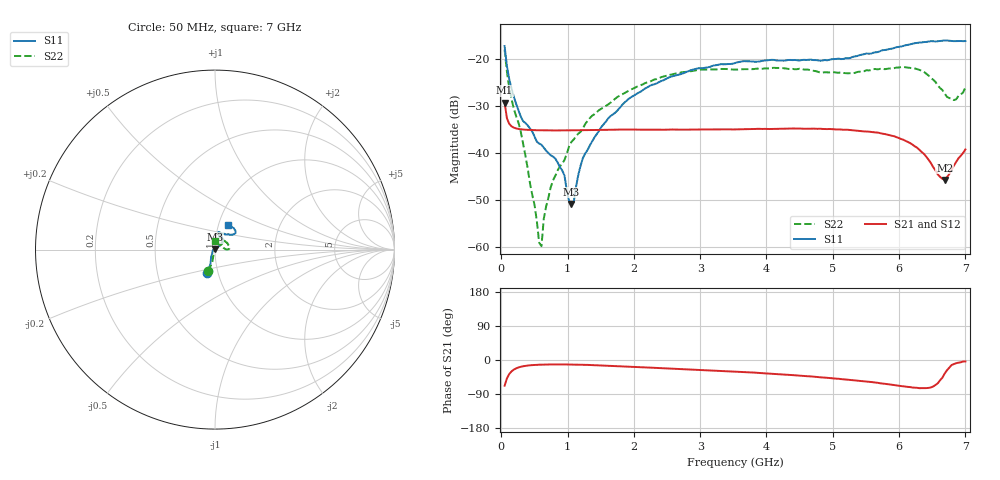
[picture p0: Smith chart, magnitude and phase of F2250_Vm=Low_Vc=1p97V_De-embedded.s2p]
! Integrated Device Technology
! Corporate Headquarters
! 6024 Silver Creek Valley Road
! San Jose, CA 95138  USA
! Phone:  1-408-284-8200
! Toll Free:  1-800-223-1366
! Webpage:  http://www.idt.com/
! Timing and RF Division
! 515 Groton Road, Suite 102
! Westford, MA 01886-6024
! Device:  F2250
! Description: Voltage Variable RF Attenuator
! Frequency:  50.0 -  6000.00 MHz
! Package:  3x3 mm Thin QFN Plastic Package: 16 pin
! Ports:  2 RF, 3 DC
!  Pin  1  = GND
!  Pin  2  = NC
!  Pin  3  = RF1  = Port 1
!  Pin  4  = NC
!  Pin  5  = GND
!  Pin  6  = GND
!  Pin  7  = GND
!  Pin  8  = GND
!  Pin  9  = NC
!  Pin 10  = RF2  = Port 2
!  Pin 11  = NC
!  Pin 12  = GND
!  Pin 13  = GND
!  Pin 14  = VCNTRL
!  Pin 15  = VDD
!  Pin 16  = VMODE
! Vcntrl:  1.970 Volts
! Vmode:  +0.000 Volts
! Vdd:  +3.30  Volts
! Current:  1.185 mA
! Data:  The device was measured on a the F2250 evaluation board which has
!  individual transmission lines to the RF pins.  Data was collected
!  using a calibrated network analyzer.  The evaluation board was
!  de-embedded using a TRL calibration technique.
!  The reference plane is the edge of the package pin.
! Misc:  SN 10
!  Action Tracker AT0258
! Date Measured:  2014-11-26
! Date:  2015-10-15  MJV
! Note:
!  Integrated Device Technology supplies this data as a sample of measured
!  data at the package pin for this product.  Your particular data for this
!  product may vary.
!  Data was taken at 25 degrees C.
!  Integrated Device Technology reserves the right to change this data at anytime.
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# GHz S dB R 50
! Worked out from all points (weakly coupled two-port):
!   201 points, 50 MHz to 7 GHz, reference 50 ohm
!   highest |S21| = -29.23 dB at 50 MHz (marker M1); lowest = -45.8 dB at 6.687 GHz (marker M2)
!   lowest |S11| = -50.9 dB at 1.058 GHz (marker M3), VSWR 1.01, Z = 49.8 + j0.242 ohm
!   |S11| at or under -10 dB: start of sweep to end of sweep
!   |S22| runs from -59.9 to -17.9 dB; largest |S21 - S12| = 5.7e-05
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0.05  -17.18 -108.6  -29.23 -67.8  -29.23 -67.8  -17.93 -107.7
0.1195  -24.20 -111.7  -33.77 -37.1  -33.77 -37.1  -26.01 -103.7
0.29325  -32.20 -127.5  -34.94 -17.9  -34.94 -17.9  -35.42 -103.6
0.50175  -36.50 -149.7  -35.12 -13.0  -35.12 -13.0  -51.09 -133.7
0.57125  -37.98 -160.3  -35.15 -12.4  -35.14 -12.4  -59.13 -177.4
0.606  -38.23 -160.9  -35.15 -12.2  -35.15 -12.2  -59.87 110.0
0.64075  -38.84 -161.1  -35.16 -12.1  -35.16 -12.0  -54.04 75.6
0.745  -40.48 -174.8  -35.17 -11.8  -35.17 -11.7  -47.34 61.6
0.9535  -44.82 169.7  -35.18 -11.7  -35.19 -11.8  -41.47 61.2
1.023  -50.29 143.2  -35.17 -11.9  -35.18 -11.9  -38.59 52.1
1.05775  -50.88 121.8  -35.17 -11.9  -35.17 -11.9  -37.64 51.3
1.0925  -50.54 87.6  -35.16 -12.0  -35.16 -12.0  -37.10 48.2
1.2315  -41.05 43.7  -35.12 -12.5  -35.12 -12.5  -34.74 38.0
1.61375  -32.60 40.7  -35.05 -15.0  -35.04 -15.0  -29.62 40.3
2.37825  -24.88 47.3  -35.01 -21.2  -35.01 -21.2  -24.06 44.0
3.525  -20.81 72.4  -34.96 -30.8  -34.97 -30.7  -22.21 67.8
4.7065  -20.18 72.3  -34.80 -43.9  -34.80 -44.0  -22.47 68.2
5.85325  -17.82 40.4  -36.18 -64.4  -36.18 -64.4  -21.97 15.9
6.33975  -16.41 40.9  -39.78 -74.2  -39.79 -74.3  -22.42 1.8
6.68725  -15.99 48.8  -45.75 -35.8  -45.74 -35.7  -27.33 22.1
6.82625  -16.14 53.6  -42.68 -10.7  -42.63 -10.8  -28.70 52.4
7  -16.12 63.2  -39.24 -3.8  -39.20 -3.9  -26.01 88.5
